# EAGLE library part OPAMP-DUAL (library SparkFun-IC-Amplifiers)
Generic op-amp footprint This component is for the standard 358 pinning of a dual op-amp From the LM358 datasheet: Pin 1: Output A Pin 2: Inverting Input A Pin 3: Non-Inverting Input A Pin 4: Gnd Pin 5: Non-Inverting Input B Pin 6: Inverting Input B Pin 7: Output B Pin 8: V+
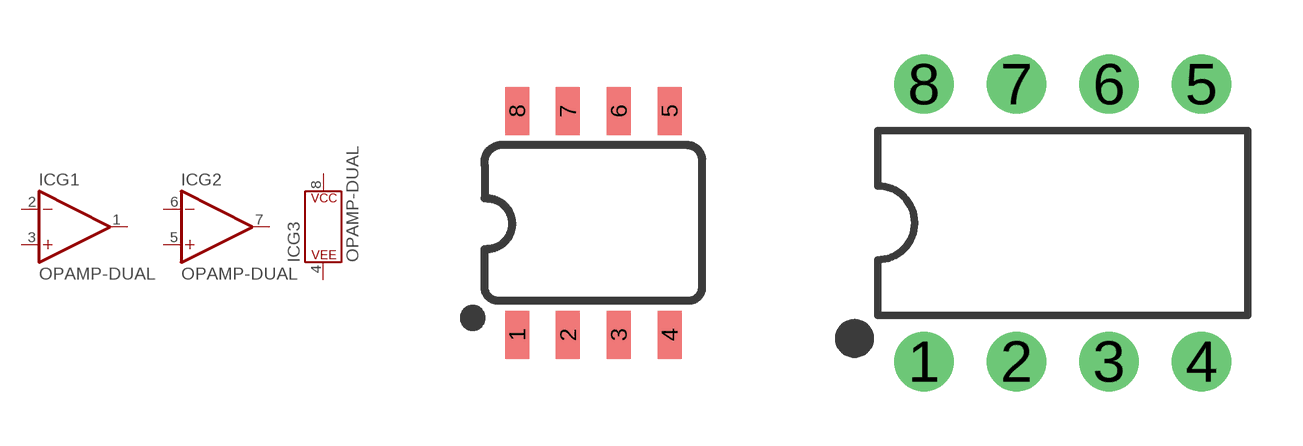
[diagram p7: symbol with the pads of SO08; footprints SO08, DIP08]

Designator prefix IC; gates G1=OP-AMP G2=OP-AMP G3=POWER_CONSORT

## OPAMP-DUALU (PROD_ID: NA-XXXXX; VALUE: OP-AMP)  [SO08]
1  G1:OUT  out
2  G1:-IN  in
3  G1:+IN  in
4  G3:P$V-
5  G2:+IN  in
6  G2:-IN  in
7  G2:OUT  out
8  G3:P$V+

## OPAMP-DUALDIP (PROD_ID: NA-XXXXX; VALUE: OP-AMP)  [DIP08]
Pads as for SO08

## Footprint SO08 (pad centres in mm)
SOIC, 0.15 inch width
smd 0.6 x 1.2: 1 -1.905,-2.8; 2 -0.635,-2.8; 3 0.635,-2.8; 4 1.905,-2.8; 5 1.905,2.8; 6 0.635,2.8; 7 -0.635,2.8; 8 -1.905,2.8

## Footprint DIP08 (pad centres in mm)
Dual In Line Package
drill 0.813 pad 1.626: 1 -3.81,-3.81; 2 -1.27,-3.81; 3 1.27,-3.81; 4 3.81,-3.81; 5 3.81,3.81; 6 1.27,3.81; 7 -1.27,3.81; 8 -3.81,3.81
